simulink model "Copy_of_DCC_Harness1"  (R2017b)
settings: Solver=FixedStepDiscrete  StartTime=0.0  StopTime=2  FixedStep=0.01  RelTol=1e-3  EnableMultiTasking=on
undefined symbols (not defined in the file): sigbuilder_block

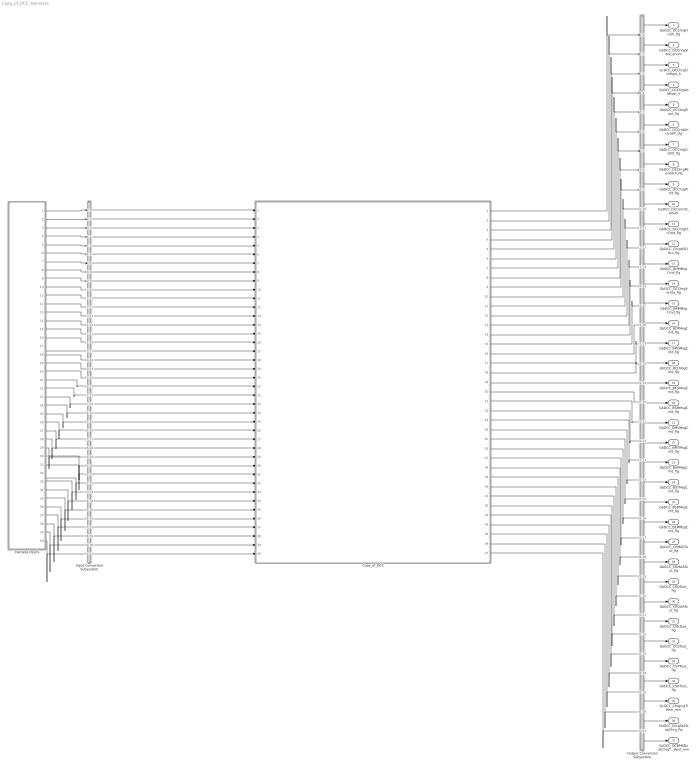
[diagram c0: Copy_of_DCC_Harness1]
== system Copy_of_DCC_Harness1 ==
  Copy_of_DCC : ModelReference  ModelNameDialog=Copy_of_DCC  SimulationMode=Normal  ModelReferenceVersion='M112C107'
  Harness Inputs : Subsystem  Tag=STV Subsys  LoadFcn=sigbuilder_block('load');  StartFcn=sigbuilder_block('start');  StopFcn=sigbuilder_block('stop');  ClipboardFcn=sigbuilder_block('clipboard');  mask(Sigbuilder block){tuvar=[0:10]}
      mask init:
      | if ~strcmp(get_param(bdroot(gcb),'SimulationStatus'),'stopped'),tuvar = sigbuilder_block('maskInit'); end
  Input Conversion Subsystem : Subsystem  Tag=__SLT_ICS__  Description=Signal spec. and routing
  Output Conversion Subsystem : Subsystem  Tag=__SLT_OCS__  Description=Signal spec. and routing
  GbDCC_DCChrgFinish_flg : Outport  OutDataTypeStr=boolean  PortDimensions=[1]
  GeDCC_DCChrgState_enum : Outport  Port=2  OutDataTypeStr=uint8  PortDimensions=[1]
  GcDCC_DCChrgCrntRqst_A : Outport  Port=3  OutDataTypeStr=single  PortDimensions=[1]
  GcDCC_DCChrgVoltRqst_V : Outport  Port=4  OutDataTypeStr=single  PortDimensions=[1]
  GbDCC_DCChrgRqst_flg : Outport  Port=5  OutDataTypeStr=boolean  PortDimensions=[1]
  GbDCC_DCCrntUnctrolFlt_flg : Outport  Port=6  OutDataTypeStr=boolean  PortDimensions=[1]
  GbDCC_DCChrgCrntFlt_flg : Outport  Port=7  OutDataTypeStr=boolean  PortDimensions=[1]
  GbDCC_DCChrgMismatch_flg : Outport  Port=8  OutDataTypeStr=boolean  PortDimensions=[1]
  GbDCC_DCChrgPrmt_flg : Outport  Port=9  OutDataTypeStr=boolean  PortDimensions=[1]
  GeDCC_DCConnSt_enum : Outport  Port=10  OutDataTypeStr=uint8  PortDimensions=[1]
  GbDCC_DCChrgCtrCmd_flg : Outport  Port=11  OutDataTypeStr=boolean  PortDimensions=[1]
  GbDCC_ChrgrISOAcv_flg : Outport  Port=12  OutDataTypeStr=boolean  PortDimensions=[1]
  GbDCC_BHMMsgCmd_flg : Outport  Port=13  OutDataTypeStr=boolean  PortDimensions=[1]
  GbDCC_DCChrgVerSta_flg : Outport  Port=14  OutDataTypeStr=boolean  PortDimensions=[1]
  GbDCC_BRMMsgCmd_flg : Outport  Port=15  OutDataTypeStr=boolean  PortDimensions=[1]
  GbDCC_BCPMsgCmd_flg : Outport  Port=16  OutDataTypeStr=boolean  PortDimensions=[1]
  GbDCC_BROMsgCmd_flg : Outport  Port=17  OutDataTypeStr=boolean  PortDimensions=[1]
  GbDCC_BCLMsgCmd_flg : Outport  Port=18  OutDataTypeStr=boolean  PortDimensions=[1]
  GbDCC_BCSMsgCmd_flg : Outport  Port=19  OutDataTypeStr=boolean  PortDimensions=[1]
  GbDCC_BSMMsgCmd_flg : Outport  Port=20  OutDataTypeStr=boolean  PortDimensions=[1]
  GbDCC_BMVMsgCmd_flg : Outport  Port=21  OutDataTypeStr=boolean  PortDimensions=[1]
  GbDCC_BMTMsgCmd_flg : Outport  Port=22  OutDataTypeStr=boolean  PortDimensions=[1]
  GbDCC_BSPMsgCmd_flg : Outport  Port=23  OutDataTypeStr=boolean  PortDimensions=[1]
  GbDCC_BSTMsgCmd_flg : Outport  Port=24  OutDataTypeStr=boolean  PortDimensions=[1]
  GbDCC_BSDMsgCmd_flg : Outport  Port=25  OutDataTypeStr=boolean  PortDimensions=[1]
  GbDCC_BEMMsgCmd_flg : Outport  Port=26  OutDataTypeStr=boolean  PortDimensions=[1]
  GbDCC_CRM00Tout_flg : Outport  Port=27  OutDataTypeStr=boolean  PortDimensions=[1]
  GbDCC_CRMAATout_flg : Outport  Port=28  OutDataTypeStr=boolean  PortDimensions=[1]
  GbDCC_CROTout_flg : Outport  Port=29  OutDataTypeStr=boolean  PortDimensions=[1]
  GbDCC_CROAATout_flg : Outport  Port=30  OutDataTypeStr=boolean  PortDimensions=[1]
  GbDCC_CMLTout_flg : Outport  Port=31  OutDataTypeStr=boolean  PortDimensions=[1]
  GbDCC_CCSTout_flg : Outport  Port=32  OutDataTypeStr=boolean  PortDimensions=[1]
  GbDCC_CSTTout_flg : Outport  Port=33  OutDataTypeStr=boolean  PortDimensions=[1]
  GbDCC_CSDTout_flg : Outport  Port=34  OutDataTypeStr=boolean  PortDimensions=[1]
  GcDCC_ChrgingTiRem_min : Outport  Port=35  OutDataTypeStr=uint16  PortDimensions=[1]
  GbDCC_ChrgSt2StepChrg_flg : Outport  Port=36  OutDataTypeStr=boolean  PortDimensions=[1]
  GcDCC_DCBMSBulkChrgTimeRest_min : Outport  Port=37  OutDataTypeStr=uint16  PortDimensions=[1]
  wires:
  Harness Inputs/1(GbGDP_CRMMsgUpd_flg) -> Input Conversion Subsystem/1(Inport_1)
  Harness Inputs/2(GbGDP_CCSMsgUpd_flg) -> Input Conversion Subsystem/2(Inport_2)
  Harness Inputs/3(GeBTM_HeatReq_enum) -> Input Conversion Subsystem/3(Inport_3)
  Harness Inputs/4(GeMSM_BMUState_enum) -> Input Conversion Subsystem/4(Inport_4)
  Harness Inputs/5(GeFTC_FltLevel_enum) -> Input Conversion Subsystem/5(Inport_5)
  Harness Inputs/6(GeCTC_CtrCtlState_enum) -> Input Conversion Subsystem/6(Inport_6)
  Harness Inputs/7(GeCTC_CtrCtlConnMode_enum) -> Input Conversion Subsystem/7(Inport_7)
  Harness Inputs/8(GbLDP_DC12VSply_flg) -> Input Conversion Subsystem/8(Inport_8)
  Harness Inputs/9(GeLDP_CC2St_enum) -> Input Conversion Subsystem/9(Inport_9)
  Harness Inputs/10(GcSOP_MaxChrgCurr_A) -> Input Conversion Subsystem/10(Inport_10)
  Harness Inputs/11(GcCDP_MaxCellVolt_mV) -> Input Conversion Subsystem/11(Inport_11)
  Harness Inputs/12(GcCDP_MinCellTemp_C) -> Input Conversion Subsystem/12(Inport_12)
  Harness Inputs/13(GcGDP_CRMChrgrAck_numb) -> Input Conversion Subsystem/13(Inport_13)
  Harness Inputs/14(GcGDP_CMLChrgrMaxVolt_V) -> Input Conversion Subsystem/14(Inport_14)
  Harness Inputs/15(GcGDP_CMLCurMaxOut_A) -> Input Conversion Subsystem/15(Inport_15)
  Harness Inputs/16(GcGDP_CROChrgrRdy_numb) -> Input Conversion Subsystem/16(Inport_16)
  Harness Inputs/17(GcGDP_CCSCurOut_A) -> Input Conversion Subsystem/17(Inport_17)
  Harness Inputs/18(GbGDP_CCSRecOnce_flg) -> Input Conversion Subsystem/18(Inport_18)
  Harness Inputs/19(GbGDP_CEMRecOnce_flg) -> Input Conversion Subsystem/19(Inport_19)
  Harness Inputs/20(GbGDP_CHMRecOnce_flg) -> Input Conversion Subsystem/20(Inport_20)
  Harness Inputs/21(GbGDP_CMLRecOnce_flg) -> Input Conversion Subsystem/21(Inport_21)
  Harness Inputs/22(GbGDP_CRMRecOnce_flg) -> Input Conversion Subsystem/22(Inport_22)
  Harness Inputs/23(GbGDP_CRORecOnce_flg) -> Input Conversion Subsystem/23(Inport_23)
  Harness Inputs/24(GbGDP_CSDRecOnce_flg) -> Input Conversion Subsystem/24(Inport_24)
  Harness Inputs/25(GbGDP_CSTRecOnce_flg) -> Input Conversion Subsystem/25(Inport_25)
  Harness Inputs/26(GbGDP_CTSRecOnce_flg) -> Input Conversion Subsystem/26(Inport_26)
  Harness Inputs/27(GcVDP_ChrgLdReq_numb) -> Input Conversion Subsystem/27(Inport_27)
  Harness Inputs/28(GeVDP_ChrgRqst_enum) -> Input Conversion Subsystem/28(Inport_28)
  Harness Inputs/29(GcHDP_PackCrnt_A) -> Input Conversion Subsystem/29(Inport_29)
  Harness Inputs/30(GcHDP_PackVolt_V) -> Input Conversion Subsystem/30(Inport_30)
  Harness Inputs/31(GcADP_VehSpd_kmh) -> Input Conversion Subsystem/31(Inport_31)
  Harness Inputs/32(GcDCS_2829Da_numb) -> Input Conversion Subsystem/32(Inport_32)
  Harness Inputs/33(GcSOC_DispSOC_pct) -> Input Conversion Subsystem/33(Inport_33)
  Harness Inputs/34(GbFTC_OpenContactor_flg) -> Input Conversion Subsystem/34(Inport_34)
  Harness Inputs/35(GbFTC_PowerDown_flg) -> Input Conversion Subsystem/35(Inport_35)
  Harness Inputs/36(GbVDP_VcuChrgDisable_flg) -> Input Conversion Subsystem/36(Inport_36)
  Harness Inputs/37(GeVDP_VcuFalutLvl_enum) -> Input Conversion Subsystem/37(Inport_37)
  Harness Inputs/38(GcUDS_FullChrgCutoffVolt_mV) -> Input Conversion Subsystem/38(Inport_38)
  Harness Inputs/39(GcCDP_MaxCellTemp_C) -> Input Conversion Subsystem/39(Inport_39)
  Harness Inputs/40(GeUDS_CapSel_enum) -> Input Conversion Subsystem/40(Inport_40)
  Output Conversion Subsystem/1(Outport_1) -> GbDCC_DCChrgFinish_flg/1
  Output Conversion Subsystem/2(Outport_2) -> GeDCC_DCChrgState_enum/1
  Output Conversion Subsystem/3(Outport_3) -> GcDCC_DCChrgCrntRqst_A/1
  Output Conversion Subsystem/4(Outport_4) -> GcDCC_DCChrgVoltRqst_V/1
  Output Conversion Subsystem/5(Outport_5) -> GbDCC_DCChrgRqst_flg/1
  Output Conversion Subsystem/6(Outport_6) -> GbDCC_DCCrntUnctrolFlt_flg/1
  Output Conversion Subsystem/7(Outport_7) -> GbDCC_DCChrgCrntFlt_flg/1
  Output Conversion Subsystem/8(Outport_8) -> GbDCC_DCChrgMismatch_flg/1
  Output Conversion Subsystem/9(Outport_9) -> GbDCC_DCChrgPrmt_flg/1
  Output Conversion Subsystem/10(Outport_10) -> GeDCC_DCConnSt_enum/1
  Output Conversion Subsystem/11(Outport_11) -> GbDCC_DCChrgCtrCmd_flg/1
  Output Conversion Subsystem/12(Outport_12) -> GbDCC_ChrgrISOAcv_flg/1
  Output Conversion Subsystem/13(Outport_13) -> GbDCC_BHMMsgCmd_flg/1
  Output Conversion Subsystem/14(Outport_14) -> GbDCC_DCChrgVerSta_flg/1
  Output Conversion Subsystem/15(Outport_15) -> GbDCC_BRMMsgCmd_flg/1
  Output Conversion Subsystem/16(Outport_16) -> GbDCC_BCPMsgCmd_flg/1
  Output Conversion Subsystem/17(Outport_17) -> GbDCC_BROMsgCmd_flg/1
  Output Conversion Subsystem/18(Outport_18) -> GbDCC_BCLMsgCmd_flg/1
  Output Conversion Subsystem/19(Outport_19) -> GbDCC_BCSMsgCmd_flg/1
  Output Conversion Subsystem/20(Outport_20) -> GbDCC_BSMMsgCmd_flg/1
  Output Conversion Subsystem/21(Outport_21) -> GbDCC_BMVMsgCmd_flg/1
  Output Conversion Subsystem/22(Outport_22) -> GbDCC_BMTMsgCmd_flg/1
  Output Conversion Subsystem/23(Outport_23) -> GbDCC_BSPMsgCmd_flg/1
  Output Conversion Subsystem/24(Outport_24) -> GbDCC_BSTMsgCmd_flg/1
  Output Conversion Subsystem/25(Outport_25) -> GbDCC_BSDMsgCmd_flg/1
  Output Conversion Subsystem/26(Outport_26) -> GbDCC_BEMMsgCmd_flg/1
  Output Conversion Subsystem/27(Outport_27) -> GbDCC_CRM00Tout_flg/1
  Output Conversion Subsystem/28(Outport_28) -> GbDCC_CRMAATout_flg/1
  Output Conversion Subsystem/29(Outport_29) -> GbDCC_CROTout_flg/1
  Output Conversion Subsystem/30(Outport_30) -> GbDCC_CROAATout_flg/1
  Output Conversion Subsystem/31(Outport_31) -> GbDCC_CMLTout_flg/1
  Output Conversion Subsystem/32(Outport_32) -> GbDCC_CCSTout_flg/1
  Output Conversion Subsystem/33(Outport_33) -> GbDCC_CSTTout_flg/1
  Output Conversion Subsystem/34(Outport_34) -> GbDCC_CSDTout_flg/1
  Output Conversion Subsystem/35(Outport_35) -> GcDCC_ChrgingTiRem_min/1
  Output Conversion Subsystem/36(Outport_36) -> GbDCC_ChrgSt2StepChrg_flg/1
  Output Conversion Subsystem/37(Outport_37) -> GcDCC_DCBMSBulkChrgTimeRest_min/1
  Input Conversion Subsystem/1(Outport_1) -> Copy_of_DCC/1
  Input Conversion Subsystem/2(Outport_2) -> Copy_of_DCC/2
  Input Conversion Subsystem/3(Outport_3) -> Copy_of_DCC/3
  Input Conversion Subsystem/4(Outport_4) -> Copy_of_DCC/4
  Input Conversion Subsystem/5(Outport_5) -> Copy_of_DCC/5
  Input Conversion Subsystem/6(Outport_6) -> Copy_of_DCC/6
  Input Conversion Subsystem/7(Outport_7) -> Copy_of_DCC/7
  Input Conversion Subsystem/8(Outport_8) -> Copy_of_DCC/8
  Input Conversion Subsystem/9(Outport_9) -> Copy_of_DCC/9
  Input Conversion Subsystem/10(Outport_10) -> Copy_of_DCC/10
  Input Conversion Subsystem/11(Outport_11) -> Copy_of_DCC/11
  Input Conversion Subsystem/12(Outport_12) -> Copy_of_DCC/12
  Input Conversion Subsystem/13(Outport_13) -> Copy_of_DCC/13
  Input Conversion Subsystem/14(Outport_14) -> Copy_of_DCC/14
  Input Conversion Subsystem/15(Outport_15) -> Copy_of_DCC/15
  Input Conversion Subsystem/16(Outport_16) -> Copy_of_DCC/16
  Input Conversion Subsystem/17(Outport_17) -> Copy_of_DCC/17
  Input Conversion Subsystem/18(Outport_18) -> Copy_of_DCC/18
  Input Conversion Subsystem/19(Outport_19) -> Copy_of_DCC/19
  Input Conversion Subsystem/20(Outport_20) -> Copy_of_DCC/20
  Input Conversion Subsystem/21(Outport_21) -> Copy_of_DCC/21
  Input Conversion Subsystem/22(Outport_22) -> Copy_of_DCC/22
  Input Conversion Subsystem/23(Outport_23) -> Copy_of_DCC/23
  Input Conversion Subsystem/24(Outport_24) -> Copy_of_DCC/24
  Input Conversion Subsystem/25(Outport_25) -> Copy_of_DCC/25
  Input Conversion Subsystem/26(Outport_26) -> Copy_of_DCC/26
  Input Conversion Subsystem/27(Outport_27) -> Copy_of_DCC/27
  Input Conversion Subsystem/28(Outport_28) -> Copy_of_DCC/28
  Input Conversion Subsystem/29(Outport_29) -> Copy_of_DCC/29
  Input Conversion Subsystem/30(Outport_30) -> Copy_of_DCC/30
  Input Conversion Subsystem/31(Outport_31) -> Copy_of_DCC/31
  Input Conversion Subsystem/32(Outport_32) -> Copy_of_DCC/32
  Input Conversion Subsystem/33(Outport_33) -> Copy_of_DCC/33
  Input Conversion Subsystem/34(Outport_34) -> Copy_of_DCC/34
  Input Conversion Subsystem/35(Outport_35) -> Copy_of_DCC/35
  Input Conversion Subsystem/36(Outport_36) -> Copy_of_DCC/36
  Input Conversion Subsystem/37(Outport_37) -> Copy_of_DCC/37
  Input Conversion Subsystem/38(Outport_38) -> Copy_of_DCC/38
  Input Conversion Subsystem/39(Outport_39) -> Copy_of_DCC/39
  Input Conversion Subsystem/40(Outport_40) -> Copy_of_DCC/40
  Copy_of_DCC/1 -> Output Conversion Subsystem/1(Inport_1)
  Copy_of_DCC/2 -> Output Conversion Subsystem/2(Inport_2)
  Copy_of_DCC/3 -> Output Conversion Subsystem/3(Inport_3)
  Copy_of_DCC/4 -> Output Conversion Subsystem/4(Inport_4)
  Copy_of_DCC/5 -> Output Conversion Subsystem/5(Inport_5)
  Copy_of_DCC/6 -> Output Conversion Subsystem/6(Inport_6)
  Copy_of_DCC/7 -> Output Conversion Subsystem/7(Inport_7)
  Copy_of_DCC/8 -> Output Conversion Subsystem/8(Inport_8)
  Copy_of_DCC/9 -> Output Conversion Subsystem/9(Inport_9)
  Copy_of_DCC/10 -> Output Conversion Subsystem/10(Inport_10)
  Copy_of_DCC/11 -> Output Conversion Subsystem/11(Inport_11)
  Copy_of_DCC/12 -> Output Conversion Subsystem/12(Inport_12)
  Copy_of_DCC/13 -> Output Conversion Subsystem/13(Inport_13)
  Copy_of_DCC/14 -> Output Conversion Subsystem/14(Inport_14)
  Copy_of_DCC/15 -> Output Conversion Subsystem/15(Inport_15)
  Copy_of_DCC/16 -> Output Conversion Subsystem/16(Inport_16)
  Copy_of_DCC/17 -> Output Conversion Subsystem/17(Inport_17)
  Copy_of_DCC/18 -> Output Conversion Subsystem/18(Inport_18)
  Copy_of_DCC/19 -> Output Conversion Subsystem/19(Inport_19)
  Copy_of_DCC/20 -> Output Conversion Subsystem/20(Inport_20)
  Copy_of_DCC/21 -> Output Conversion Subsystem/21(Inport_21)
  Copy_of_DCC/22 -> Output Conversion Subsystem/22(Inport_22)
  Copy_of_DCC/23 -> Output Conversion Subsystem/23(Inport_23)
  Copy_of_DCC/24 -> Output Conversion Subsystem/24(Inport_24)
  Copy_of_DCC/25 -> Output Conversion Subsystem/25(Inport_25)
  Copy_of_DCC/26 -> Output Conversion Subsystem/26(Inport_26)
  Copy_of_DCC/27 -> Output Conversion Subsystem/27(Inport_27)
  Copy_of_DCC/28 -> Output Conversion Subsystem/28(Inport_28)
  Copy_of_DCC/29 -> Output Conversion Subsystem/29(Inport_29)
  Copy_of_DCC/30 -> Output Conversion Subsystem/30(Inport_30)
  Copy_of_DCC/31 -> Output Conversion Subsystem/31(Inport_31)
  Copy_of_DCC/32 -> Output Conversion Subsystem/32(Inport_32)
  Copy_of_DCC/33 -> Output Conversion Subsystem/33(Inport_33)
  Copy_of_DCC/34 -> Output Conversion Subsystem/34(Inport_34)
  Copy_of_DCC/35 -> Output Conversion Subsystem/35(Inport_35)
  Copy_of_DCC/36 -> Output Conversion Subsystem/36(Inport_36)
  Copy_of_DCC/37 -> Output Conversion Subsystem/37(Inport_37)

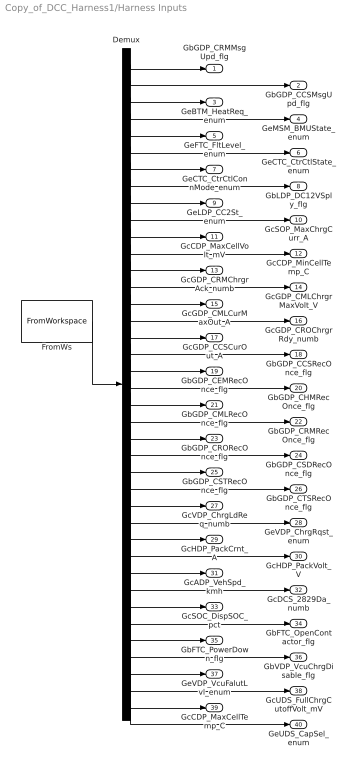
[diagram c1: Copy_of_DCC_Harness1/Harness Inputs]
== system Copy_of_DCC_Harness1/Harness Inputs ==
  Demux : Demux  Tag=STV Demux  Outputs=40
  FromWs : FromWorkspace  Tag=STV FromWs  VariableName=tuvar  SampleTime=0
  GbGDP_CRMMsgUpd_flg : Outport  Tag=STV Outport
  GbGDP_CCSMsgUpd_flg : Outport  Tag=STV Outport  Port=2
  GeBTM_HeatReq_enum : Outport  Tag=STV Outport  Port=3
  GeMSM_BMUState_enum : Outport  Tag=STV Outport  Port=4
  GeFTC_FltLevel_enum : Outport  Tag=STV Outport  Port=5
  GeCTC_CtrCtlState_enum : Outport  Tag=STV Outport  Port=6
  GeCTC_CtrCtlConnMode_enum : Outport  Tag=STV Outport  Port=7
  GbLDP_DC12VSply_flg : Outport  Tag=STV Outport  Port=8
  GeLDP_CC2St_enum : Outport  Tag=STV Outport  Port=9
  GcSOP_MaxChrgCurr_A : Outport  Tag=STV Outport  Port=10
  GcCDP_MaxCellVolt_mV : Outport  Tag=STV Outport  Port=11
  GcCDP_MinCellTemp_C : Outport  Tag=STV Outport  Port=12
  GcGDP_CRMChrgrAck_numb : Outport  Tag=STV Outport  Port=13
  GcGDP_CMLChrgrMaxVolt_V : Outport  Tag=STV Outport  Port=14
  GcGDP_CMLCurMaxOut_A : Outport  Tag=STV Outport  Port=15
  GcGDP_CROChrgrRdy_numb : Outport  Tag=STV Outport  Port=16
  GcGDP_CCSCurOut_A : Outport  Tag=STV Outport  Port=17
  GbGDP_CCSRecOnce_flg : Outport  Tag=STV Outport  Port=18
  GbGDP_CEMRecOnce_flg : Outport  Tag=STV Outport  Port=19
  GbGDP_CHMRecOnce_flg : Outport  Tag=STV Outport  Port=20
  GbGDP_CMLRecOnce_flg : Outport  Tag=STV Outport  Port=21
  GbGDP_CRMRecOnce_flg : Outport  Tag=STV Outport  Port=22
  GbGDP_CRORecOnce_flg : Outport  Tag=STV Outport  Port=23
  GbGDP_CSDRecOnce_flg : Outport  Tag=STV Outport  Port=24
  GbGDP_CSTRecOnce_flg : Outport  Tag=STV Outport  Port=25
  GbGDP_CTSRecOnce_flg : Outport  Tag=STV Outport  Port=26
  GcVDP_ChrgLdReq_numb : Outport  Tag=STV Outport  Port=27
  GeVDP_ChrgRqst_enum : Outport  Tag=STV Outport  Port=28
  GcHDP_PackCrnt_A : Outport  Tag=STV Outport  Port=29
  GcHDP_PackVolt_V : Outport  Tag=STV Outport  Port=30
  GcADP_VehSpd_kmh : Outport  Tag=STV Outport  Port=31
  GcDCS_2829Da_numb : Outport  Tag=STV Outport  Port=32
  GcSOC_DispSOC_pct : Outport  Tag=STV Outport  Port=33
  GbFTC_OpenContactor_flg : Outport  Tag=STV Outport  Port=34
  GbFTC_PowerDown_flg : Outport  Tag=STV Outport  Port=35
  GbVDP_VcuChrgDisable_flg : Outport  Tag=STV Outport  Port=36
  GeVDP_VcuFalutLvl_enum : Outport  Tag=STV Outport  Port=37
  GcUDS_FullChrgCutoffVolt_mV : Outport  Tag=STV Outport  Port=38
  GcCDP_MaxCellTemp_C : Outport  Tag=STV Outport  Port=39
  GeUDS_CapSel_enum : Outport  Tag=STV Outport  Port=40
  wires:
  FromWs/1 -> Demux/1
  Demux/1 -> GbGDP_CRMMsgUpd_flg/1
  Demux/2 -> GbGDP_CCSMsgUpd_flg/1
  Demux/3 -> GeBTM_HeatReq_enum/1
  Demux/4 -> GeMSM_BMUState_enum/1
  Demux/5 -> GeFTC_FltLevel_enum/1
  Demux/6 -> GeCTC_CtrCtlState_enum/1
  Demux/7 -> GeCTC_CtrCtlConnMode_enum/1
  Demux/8 -> GbLDP_DC12VSply_flg/1
  Demux/9 -> GeLDP_CC2St_enum/1
  Demux/10 -> GcSOP_MaxChrgCurr_A/1
  Demux/11 -> GcCDP_MaxCellVolt_mV/1
  Demux/12 -> GcCDP_MinCellTemp_C/1
  Demux/13 -> GcGDP_CRMChrgrAck_numb/1
  Demux/14 -> GcGDP_CMLChrgrMaxVolt_V/1
  Demux/15 -> GcGDP_CMLCurMaxOut_A/1
  Demux/16 -> GcGDP_CROChrgrRdy_numb/1
  Demux/17 -> GcGDP_CCSCurOut_A/1
  Demux/18 -> GbGDP_CCSRecOnce_flg/1
  Demux/19 -> GbGDP_CEMRecOnce_flg/1
  Demux/20 -> GbGDP_CHMRecOnce_flg/1
  Demux/21 -> GbGDP_CMLRecOnce_flg/1
  Demux/22 -> GbGDP_CRMRecOnce_flg/1
  Demux/23 -> GbGDP_CRORecOnce_flg/1
  Demux/24 -> GbGDP_CSDRecOnce_flg/1
  Demux/25 -> GbGDP_CSTRecOnce_flg/1
  Demux/26 -> GbGDP_CTSRecOnce_flg/1
  Demux/27 -> GcVDP_ChrgLdReq_numb/1
  Demux/28 -> GeVDP_ChrgRqst_enum/1
  Demux/29 -> GcHDP_PackCrnt_A/1
  Demux/30 -> GcHDP_PackVolt_V/1
  Demux/31 -> GcADP_VehSpd_kmh/1
  Demux/32 -> GcDCS_2829Da_numb/1
  Demux/33 -> GcSOC_DispSOC_pct/1
  Demux/34 -> GbFTC_OpenContactor_flg/1
  Demux/35 -> GbFTC_PowerDown_flg/1
  Demux/36 -> GbVDP_VcuChrgDisable_flg/1
  Demux/37 -> GeVDP_VcuFalutLvl_enum/1
  Demux/38 -> GcUDS_FullChrgCutoffVolt_mV/1
  Demux/39 -> GcCDP_MaxCellTemp_C/1
  Demux/40 -> GeUDS_CapSel_enum/1

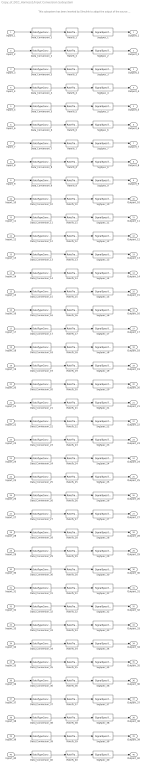
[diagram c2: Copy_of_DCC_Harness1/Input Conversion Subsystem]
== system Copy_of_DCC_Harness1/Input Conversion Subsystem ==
  note: This subsystem has been inserted by Simulink to adapt the output of the source blocks to the interface required by the harnessed component. Modifying the contents of this subsystem may result in compilation and simulation failure.
  Inport_1 : Inport
  Inport_2 : Inport  Port=2
  Inport_3 : Inport  Port=3
  Inport_4 : Inport  Port=4
  Inport_5 : Inport  Port=5
  Inport_6 : Inport  Port=6
  Inport_7 : Inport  Port=7
  Inport_8 : Inport  Port=8
  Inport_9 : Inport  Port=9
  Inport_10 : Inport  Port=10
  Inport_11 : Inport  Port=11
  Inport_12 : Inport  Port=12
  Inport_13 : Inport  Port=13
  Inport_14 : Inport  Port=14
  Inport_15 : Inport  Port=15
  Inport_16 : Inport  Port=16
  Inport_17 : Inport  Port=17
  Inport_18 : Inport  Port=18
  Inport_19 : Inport  Port=19
  Inport_20 : Inport  Port=20
  Inport_21 : Inport  Port=21
  Inport_22 : Inport  Port=22
  Inport_23 : Inport  Port=23
  Inport_24 : Inport  Port=24
  Inport_25 : Inport  Port=25
  Inport_26 : Inport  Port=26
  Inport_27 : Inport  Port=27
  Inport_28 : Inport  Port=28
  Inport_29 : Inport  Port=29
  Inport_30 : Inport  Port=30
  Inport_31 : Inport  Port=31
  Inport_32 : Inport  Port=32
  Inport_33 : Inport  Port=33
  Inport_34 : Inport  Port=34
  Inport_35 : Inport  Port=35
  Inport_36 : Inport  Port=36
  Inport_37 : Inport  Port=37
  Inport_38 : Inport  Port=38
  Inport_39 : Inport  Port=39
  Inport_40 : Inport  Port=40
  Data_Conversion_{1..2,8,18..26,34..36} (15 alike) : DataTypeConversion  OutDataTypeStr=boolean
  Data_Conversion_{10,12,14..15,17,27,29..31,33,39} (11 alike) : DataTypeConversion  OutDataTypeStr=single
  Data_Conversion_11 : DataTypeConversion  OutDataTypeStr=uint16
  Data_Conversion_{3..7,9,13,16,28,32,37,40} (12 alike) : DataTypeConversion  OutDataTypeStr=uint8
  Data_Conversion_38 : DataTypeConversion  OutDataTypeStr=uint16
  RateTs_{1..40} (40 alike) : RateTransition  OutPortSampleTime=0.01
  SigSpec_{1..2,8,18..26,34..35} (14 alike) : SignalSpecification  OutDataTypeStr=boolean  Unit=flag  Dimensions=[1]  SampleTime=0.01
  SigSpec_{10,15,17,29} (4 alike) : SignalSpecification  OutDataTypeStr=single  Unit=A  Dimensions=[1]  SampleTime=0.01
  SigSpec_11 : SignalSpecification  OutDataTypeStr=uint16  Unit=mV  Dimensions=[1]  SampleTime=0.01
  SigSpec_12 : SignalSpecification  OutDataTypeStr=single  Unit=C  Dimensions=[1]  SampleTime=0.01
  SigSpec_{13,16,32,40} (4 alike) : SignalSpecification  OutDataTypeStr=uint8  Unit=numb  Dimensions=[1]  SampleTime=0.01
  SigSpec_14 : SignalSpecification  OutDataTypeStr=single  Unit=V  Dimensions=[1]  SampleTime=0.01
  SigSpec_27 : SignalSpecification  OutDataTypeStr=single  Unit=kW  Dimensions=[1]  SampleTime=0.01
  SigSpec_{3..7,9,28,37} (8 alike) : SignalSpecification  OutDataTypeStr=uint8  Unit=enum  Dimensions=[1]  SampleTime=0.01
  SigSpec_30 : SignalSpecification  OutDataTypeStr=single  Unit=V  Dimensions=[1]  SampleTime=0.01
  SigSpec_31 : SignalSpecification  OutDataTypeStr=single  Unit=Km/h  Dimensions=[1]  SampleTime=0.01
  SigSpec_33 : SignalSpecification  OutDataTypeStr=single  Unit=pct  Dimensions=[1]  SampleTime=0.01
  SigSpec_36 : SignalSpecification  OutDataTypeStr=boolean  Unit=flg  Dimensions=[1]  SampleTime=0.01
  SigSpec_38 : SignalSpecification  OutDataTypeStr=uint16  Unit=mV  Dimensions=[1]  SampleTime=0.01
  SigSpec_39 : SignalSpecification  OutDataTypeStr=single  Unit=C  Dimensions=[1]  SampleTime=0.01
  Outport_1 : Outport
  Outport_2 : Outport  Port=2
  Outport_3 : Outport  Port=3
  Outport_4 : Outport  Port=4
  Outport_5 : Outport  Port=5
  Outport_6 : Outport  Port=6
  Outport_7 : Outport  Port=7
  Outport_8 : Outport  Port=8
  Outport_9 : Outport  Port=9
  Outport_10 : Outport  Port=10
  Outport_11 : Outport  Port=11
  Outport_12 : Outport  Port=12
  Outport_13 : Outport  Port=13
  Outport_14 : Outport  Port=14
  Outport_15 : Outport  Port=15
  Outport_16 : Outport  Port=16
  Outport_17 : Outport  Port=17
  Outport_18 : Outport  Port=18
  Outport_19 : Outport  Port=19
  Outport_20 : Outport  Port=20
  Outport_21 : Outport  Port=21
  Outport_22 : Outport  Port=22
  Outport_23 : Outport  Port=23
  Outport_24 : Outport  Port=24
  Outport_25 : Outport  Port=25
  Outport_26 : Outport  Port=26
  Outport_27 : Outport  Port=27
  Outport_28 : Outport  Port=28
  Outport_29 : Outport  Port=29
  Outport_30 : Outport  Port=30
  Outport_31 : Outport  Port=31
  Outport_32 : Outport  Port=32
  Outport_33 : Outport  Port=33
  Outport_34 : Outport  Port=34
  Outport_35 : Outport  Port=35
  Outport_36 : Outport  Port=36
  Outport_37 : Outport  Port=37
  Outport_38 : Outport  Port=38
  Outport_39 : Outport  Port=39
  Outport_40 : Outport  Port=40
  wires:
  SigSpec_1/1 -> Outport_1/1
  RateTs_1/1 -> SigSpec_1/1
  Data_Conversion_1/1 -> RateTs_1/1
  Inport_1/1 -> Data_Conversion_1/1
  SigSpec_2/1 -> Outport_2/1
  RateTs_2/1 -> SigSpec_2/1
  Data_Conversion_2/1 -> RateTs_2/1
  Inport_2/1 -> Data_Conversion_2/1
  SigSpec_3/1 -> Outport_3/1
  RateTs_3/1 -> SigSpec_3/1
  Data_Conversion_3/1 -> RateTs_3/1
  Inport_3/1 -> Data_Conversion_3/1
  SigSpec_4/1 -> Outport_4/1
  RateTs_4/1 -> SigSpec_4/1
  Data_Conversion_4/1 -> RateTs_4/1
  Inport_4/1 -> Data_Conversion_4/1
  SigSpec_5/1 -> Outport_5/1
  RateTs_5/1 -> SigSpec_5/1
  Data_Conversion_5/1 -> RateTs_5/1
  Inport_5/1 -> Data_Conversion_5/1
  SigSpec_6/1 -> Outport_6/1
  RateTs_6/1 -> SigSpec_6/1
  Data_Conversion_6/1 -> RateTs_6/1
  Inport_6/1 -> Data_Conversion_6/1
  SigSpec_7/1 -> Outport_7/1
  RateTs_7/1 -> SigSpec_7/1
  Data_Conversion_7/1 -> RateTs_7/1
  Inport_7/1 -> Data_Conversion_7/1
  SigSpec_8/1 -> Outport_8/1
  RateTs_8/1 -> SigSpec_8/1
  Data_Conversion_8/1 -> RateTs_8/1
  Inport_8/1 -> Data_Conversion_8/1
  SigSpec_9/1 -> Outport_9/1
  RateTs_9/1 -> SigSpec_9/1
  Data_Conversion_9/1 -> RateTs_9/1
  Inport_9/1 -> Data_Conversion_9/1
  SigSpec_10/1 -> Outport_10/1
  RateTs_10/1 -> SigSpec_10/1
  Data_Conversion_10/1 -> RateTs_10/1
  Inport_10/1 -> Data_Conversion_10/1
  SigSpec_11/1 -> Outport_11/1
  RateTs_11/1 -> SigSpec_11/1
  Data_Conversion_11/1 -> RateTs_11/1
  Inport_11/1 -> Data_Conversion_11/1
  SigSpec_12/1 -> Outport_12/1
  RateTs_12/1 -> SigSpec_12/1
  Data_Conversion_12/1 -> RateTs_12/1
  Inport_12/1 -> Data_Conversion_12/1
  SigSpec_13/1 -> Outport_13/1
  RateTs_13/1 -> SigSpec_13/1
  Data_Conversion_13/1 -> RateTs_13/1
  Inport_13/1 -> Data_Conversion_13/1
  SigSpec_14/1 -> Outport_14/1
  RateTs_14/1 -> SigSpec_14/1
  Data_Conversion_14/1 -> RateTs_14/1
  Inport_14/1 -> Data_Conversion_14/1
  SigSpec_15/1 -> Outport_15/1
  RateTs_15/1 -> SigSpec_15/1
  Data_Conversion_15/1 -> RateTs_15/1
  Inport_15/1 -> Data_Conversion_15/1
  SigSpec_16/1 -> Outport_16/1
  RateTs_16/1 -> SigSpec_16/1
  Data_Conversion_16/1 -> RateTs_16/1
  Inport_16/1 -> Data_Conversion_16/1
  SigSpec_17/1 -> Outport_17/1
  RateTs_17/1 -> SigSpec_17/1
  Data_Conversion_17/1 -> RateTs_17/1
  Inport_17/1 -> Data_Conversion_17/1
  SigSpec_18/1 -> Outport_18/1
  RateTs_18/1 -> SigSpec_18/1
  Data_Conversion_18/1 -> RateTs_18/1
  Inport_18/1 -> Data_Conversion_18/1
  SigSpec_19/1 -> Outport_19/1
  RateTs_19/1 -> SigSpec_19/1
  Data_Conversion_19/1 -> RateTs_19/1
  Inport_19/1 -> Data_Conversion_19/1
  SigSpec_20/1 -> Outport_20/1
  RateTs_20/1 -> SigSpec_20/1
  Data_Conversion_20/1 -> RateTs_20/1
  Inport_20/1 -> Data_Conversion_20/1
  SigSpec_21/1 -> Outport_21/1
  RateTs_21/1 -> SigSpec_21/1
  Data_Conversion_21/1 -> RateTs_21/1
  Inport_21/1 -> Data_Conversion_21/1
  SigSpec_22/1 -> Outport_22/1
  RateTs_22/1 -> SigSpec_22/1
  Data_Conversion_22/1 -> RateTs_22/1
  Inport_22/1 -> Data_Conversion_22/1
  SigSpec_23/1 -> Outport_23/1
  RateTs_23/1 -> SigSpec_23/1
  Data_Conversion_23/1 -> RateTs_23/1
  Inport_23/1 -> Data_Conversion_23/1
  SigSpec_24/1 -> Outport_24/1
  RateTs_24/1 -> SigSpec_24/1
  Data_Conversion_24/1 -> RateTs_24/1
  Inport_24/1 -> Data_Conversion_24/1
  SigSpec_25/1 -> Outport_25/1
  RateTs_25/1 -> SigSpec_25/1
  Data_Conversion_25/1 -> RateTs_25/1
  Inport_25/1 -> Data_Conversion_25/1
  SigSpec_26/1 -> Outport_26/1
  RateTs_26/1 -> SigSpec_26/1
  Data_Conversion_26/1 -> RateTs_26/1
  Inport_26/1 -> Data_Conversion_26/1
  SigSpec_27/1 -> Outport_27/1
  RateTs_27/1 -> SigSpec_27/1
  Data_Conversion_27/1 -> RateTs_27/1
  Inport_27/1 -> Data_Conversion_27/1
  SigSpec_28/1 -> Outport_28/1
  RateTs_28/1 -> SigSpec_28/1
  Data_Conversion_28/1 -> RateTs_28/1
  Inport_28/1 -> Data_Conversion_28/1
  SigSpec_29/1 -> Outport_29/1
  RateTs_29/1 -> SigSpec_29/1
  Data_Conversion_29/1 -> RateTs_29/1
  Inport_29/1 -> Data_Conversion_29/1
  SigSpec_30/1 -> Outport_30/1
  RateTs_30/1 -> SigSpec_30/1
  Data_Conversion_30/1 -> RateTs_30/1
  Inport_30/1 -> Data_Conversion_30/1
  SigSpec_31/1 -> Outport_31/1
  RateTs_31/1 -> SigSpec_31/1
  Data_Conversion_31/1 -> RateTs_31/1
  Inport_31/1 -> Data_Conversion_31/1
  SigSpec_32/1 -> Outport_32/1
  RateTs_32/1 -> SigSpec_32/1
  Data_Conversion_32/1 -> RateTs_32/1
  Inport_32/1 -> Data_Conversion_32/1
  SigSpec_33/1 -> Outport_33/1
  RateTs_33/1 -> SigSpec_33/1
  Data_Conversion_33/1 -> RateTs_33/1
  Inport_33/1 -> Data_Conversion_33/1
  SigSpec_34/1 -> Outport_34/1
  RateTs_34/1 -> SigSpec_34/1
  Data_Conversion_34/1 -> RateTs_34/1
  Inport_34/1 -> Data_Conversion_34/1
  SigSpec_35/1 -> Outport_35/1
  RateTs_35/1 -> SigSpec_35/1
  Data_Conversion_35/1 -> RateTs_35/1
  Inport_35/1 -> Data_Conversion_35/1
  SigSpec_36/1 -> Outport_36/1
  RateTs_36/1 -> SigSpec_36/1
  Data_Conversion_36/1 -> RateTs_36/1
  Inport_36/1 -> Data_Conversion_36/1
  SigSpec_37/1 -> Outport_37/1
  RateTs_37/1 -> SigSpec_37/1
  Data_Conversion_37/1 -> RateTs_37/1
  Inport_37/1 -> Data_Conversion_37/1
  SigSpec_38/1 -> Outport_38/1
  RateTs_38/1 -> SigSpec_38/1
  Data_Conversion_38/1 -> RateTs_38/1
  Inport_38/1 -> Data_Conversion_38/1
  SigSpec_39/1 -> Outport_39/1
  RateTs_39/1 -> SigSpec_39/1
  Data_Conversion_39/1 -> RateTs_39/1
  Inport_39/1 -> Data_Conversion_39/1
  SigSpec_40/1 -> Outport_40/1
  RateTs_40/1 -> SigSpec_40/1
  Data_Conversion_40/1 -> RateTs_40/1
  Inport_40/1 -> Data_Conversion_40/1

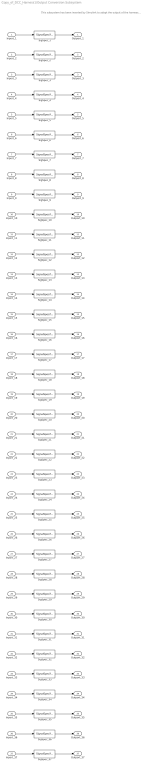
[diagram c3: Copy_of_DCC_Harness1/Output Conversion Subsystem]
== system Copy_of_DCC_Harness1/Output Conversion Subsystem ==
  note: This subsystem has been inserted by Simulink to adapt the output of the harnessed component to the interface required by the sink blocks. Modifying the contents of this subsystem may result in compilation and simulation failure.
  Inport_1 : Inport
  Inport_2 : Inport  Port=2
  Inport_3 : Inport  Port=3
  Inport_4 : Inport  Port=4
  Inport_5 : Inport  Port=5
  Inport_6 : Inport  Port=6
  Inport_7 : Inport  Port=7
  Inport_8 : Inport  Port=8
  Inport_9 : Inport  Port=9
  Inport_10 : Inport  Port=10
  Inport_11 : Inport  Port=11
  Inport_12 : Inport  Port=12
  Inport_13 : Inport  Port=13
  Inport_14 : Inport  Port=14
  Inport_15 : Inport  Port=15
  Inport_16 : Inport  Port=16
  Inport_17 : Inport  Port=17
  Inport_18 : Inport  Port=18
  Inport_19 : Inport  Port=19
  Inport_20 : Inport  Port=20
  Inport_21 : Inport  Port=21
  Inport_22 : Inport  Port=22
  Inport_23 : Inport  Port=23
  Inport_24 : Inport  Port=24
  Inport_25 : Inport  Port=25
  Inport_26 : Inport  Port=26
  Inport_27 : Inport  Port=27
  Inport_28 : Inport  Port=28
  Inport_29 : Inport  Port=29
  Inport_30 : Inport  Port=30
  Inport_31 : Inport  Port=31
  Inport_32 : Inport  Port=32
  Inport_33 : Inport  Port=33
  Inport_34 : Inport  Port=34
  Inport_35 : Inport  Port=35
  Inport_36 : Inport  Port=36
  Inport_37 : Inport  Port=37
  SigSpec_{1,5..9,11..13,15..34,36} (30 alike) : SignalSpecification  OutDataTypeStr=boolean  Unit=flag  Dimensions=[1]  SampleTime=0.01
  SigSpec_10 : SignalSpecification  OutDataTypeStr=uint8  Unit=enum  Dimensions=[1]  SampleTime=0.01
  SigSpec_14 : SignalSpecification  OutDataTypeStr=boolean  Unit=flag  Dimensions=[1]
  SigSpec_2 : SignalSpecification  OutDataTypeStr=uint8  Unit=enum  Dimensions=[1]  SampleTime=0.01
  SigSpec_3 : SignalSpecification  OutDataTypeStr=single  Unit=A  Dimensions=[1]  SampleTime=0.01
  SigSpec_35 : SignalSpecification  OutDataTypeStr=uint16  Unit=min  Dimensions=[1]  SampleTime=0.01
  SigSpec_37 : SignalSpecification  OutDataTypeStr=uint16  Unit=min  Dimensions=[1]  SampleTime=0.01
  SigSpec_4 : SignalSpecification  OutDataTypeStr=single  Unit=V  Dimensions=[1]  SampleTime=0.01
  Outport_1 : Outport
  Outport_2 : Outport  Port=2
  Outport_3 : Outport  Port=3
  Outport_4 : Outport  Port=4
  Outport_5 : Outport  Port=5
  Outport_6 : Outport  Port=6
  Outport_7 : Outport  Port=7
  Outport_8 : Outport  Port=8
  Outport_9 : Outport  Port=9
  Outport_10 : Outport  Port=10
  Outport_11 : Outport  Port=11
  Outport_12 : Outport  Port=12
  Outport_13 : Outport  Port=13
  Outport_14 : Outport  Port=14
  Outport_15 : Outport  Port=15
  Outport_16 : Outport  Port=16
  Outport_17 : Outport  Port=17
  Outport_18 : Outport  Port=18
  Outport_19 : Outport  Port=19
  Outport_20 : Outport  Port=20
  Outport_21 : Outport  Port=21
  Outport_22 : Outport  Port=22
  Outport_23 : Outport  Port=23
  Outport_24 : Outport  Port=24
  Outport_25 : Outport  Port=25
  Outport_26 : Outport  Port=26
  Outport_27 : Outport  Port=27
  Outport_28 : Outport  Port=28
  Outport_29 : Outport  Port=29
  Outport_30 : Outport  Port=30
  Outport_31 : Outport  Port=31
  Outport_32 : Outport  Port=32
  Outport_33 : Outport  Port=33
  Outport_34 : Outport  Port=34
  Outport_35 : Outport  Port=35
  Outport_36 : Outport  Port=36
  Outport_37 : Outport  Port=37
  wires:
  Inport_1/1 -> SigSpec_1/1
  SigSpec_1/1 -> Outport_1/1
  Inport_2/1 -> SigSpec_2/1
  SigSpec_2/1 -> Outport_2/1
  Inport_3/1 -> SigSpec_3/1
  SigSpec_3/1 -> Outport_3/1
  Inport_4/1 -> SigSpec_4/1
  SigSpec_4/1 -> Outport_4/1
  Inport_5/1 -> SigSpec_5/1
  SigSpec_5/1 -> Outport_5/1
  Inport_6/1 -> SigSpec_6/1
  SigSpec_6/1 -> Outport_6/1
  Inport_7/1 -> SigSpec_7/1
  SigSpec_7/1 -> Outport_7/1
  Inport_8/1 -> SigSpec_8/1
  SigSpec_8/1 -> Outport_8/1
  Inport_9/1 -> SigSpec_9/1
  SigSpec_9/1 -> Outport_9/1
  Inport_10/1 -> SigSpec_10/1
  SigSpec_10/1 -> Outport_10/1
  Inport_11/1 -> SigSpec_11/1
  SigSpec_11/1 -> Outport_11/1
  Inport_12/1 -> SigSpec_12/1
  SigSpec_12/1 -> Outport_12/1
  Inport_13/1 -> SigSpec_13/1
  SigSpec_13/1 -> Outport_13/1
  Inport_14/1 -> SigSpec_14/1
  SigSpec_14/1 -> Outport_14/1
  Inport_15/1 -> SigSpec_15/1
  SigSpec_15/1 -> Outport_15/1
  Inport_16/1 -> SigSpec_16/1
  SigSpec_16/1 -> Outport_16/1
  Inport_17/1 -> SigSpec_17/1
  SigSpec_17/1 -> Outport_17/1
  Inport_18/1 -> SigSpec_18/1
  SigSpec_18/1 -> Outport_18/1
  Inport_19/1 -> SigSpec_19/1
  SigSpec_19/1 -> Outport_19/1
  Inport_20/1 -> SigSpec_20/1
  SigSpec_20/1 -> Outport_20/1
  Inport_21/1 -> SigSpec_21/1
  SigSpec_21/1 -> Outport_21/1
  Inport_22/1 -> SigSpec_22/1
  SigSpec_22/1 -> Outport_22/1
  Inport_23/1 -> SigSpec_23/1
  SigSpec_23/1 -> Outport_23/1
  Inport_24/1 -> SigSpec_24/1
  SigSpec_24/1 -> Outport_24/1
  Inport_25/1 -> SigSpec_25/1
  SigSpec_25/1 -> Outport_25/1
  Inport_26/1 -> SigSpec_26/1
  SigSpec_26/1 -> Outport_26/1
  Inport_27/1 -> SigSpec_27/1
  SigSpec_27/1 -> Outport_27/1
  Inport_28/1 -> SigSpec_28/1
  SigSpec_28/1 -> Outport_28/1
  Inport_29/1 -> SigSpec_29/1
  SigSpec_29/1 -> Outport_29/1
  Inport_30/1 -> SigSpec_30/1
  SigSpec_30/1 -> Outport_30/1
  Inport_31/1 -> SigSpec_31/1
  SigSpec_31/1 -> Outport_31/1
  Inport_32/1 -> SigSpec_32/1
  SigSpec_32/1 -> Outport_32/1
  Inport_33/1 -> SigSpec_33/1
  SigSpec_33/1 -> Outport_33/1
  Inport_34/1 -> SigSpec_34/1
  SigSpec_34/1 -> Outport_34/1
  Inport_35/1 -> SigSpec_35/1
  SigSpec_35/1 -> Outport_35/1
  Inport_36/1 -> SigSpec_36/1
  SigSpec_36/1 -> Outport_36/1
  Inport_37/1 -> SigSpec_37/1
  SigSpec_37/1 -> Outport_37/1
